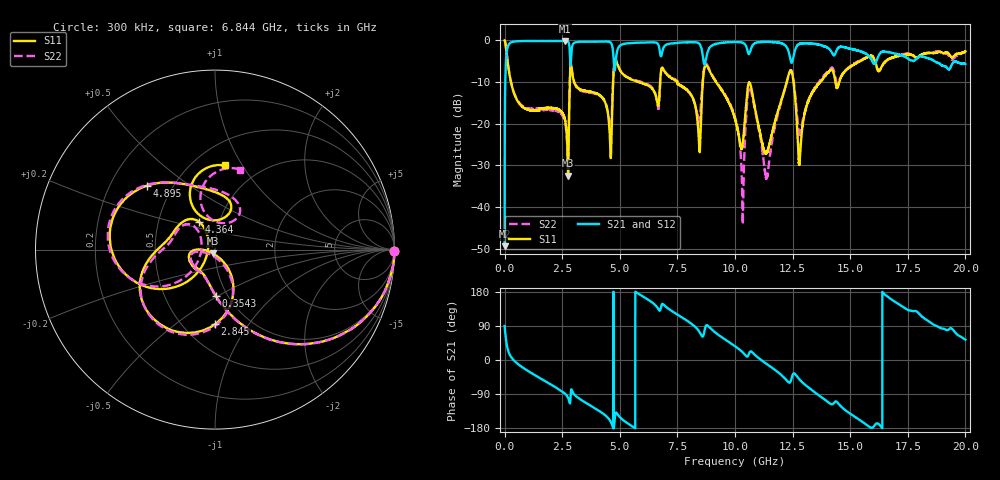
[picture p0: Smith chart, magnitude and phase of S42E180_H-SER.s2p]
!{S42E180}
!Johanson Technology Inc.
!www.johansontechnology.com
!Test Board Conditions:
!Substrate Type  RO4350B
!Substrate Thickness  50 mil
!Substrate Dk  3.66
!TL Type: GCPW
!TL Trace Width  60 mil
!TL Gap  10 mil
!Electrode orientation  Horizontal
!DUT TOPOLOGY	SERIES
!Mounting Pad LxW  14x55 mil
! Created Wed Nov 25 22:02:25 2020
# khz S ma R 50
! 2 Port Network Data from SP1.SP block
! freq  magS11  angS11  magS21  angS21  magS12  angS12  magS22  angS22
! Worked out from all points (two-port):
!   20001 points, 300 kHz to 20 GHz, reference 50 ohm
!   highest |S21| = -0.10 dB at 2.609 GHz (marker M1); lowest = -49.4 dB at 300 kHz (marker M2)
!   |S21| within 3 dB of the highest: 86.64 MHz to 2.834 GHz (2.747 GHz wide, 188 % of centre); 4.862 GHz to 6.751 GHz (1.889 GHz wide, 32.5 % of centre)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
!   lowest |S11| = -32.5 dB at 2.757 GHz (marker M3), VSWR 1.05, Z = 48.9 - j2.08 ohm
!   |S11| at or under -10 dB: 276.1 MHz to 2.831 GHz (2.555 GHz wide, 164 % of centre); 3.024 GHz to 4.71 GHz (1.687 GHz wide, 43.6 % of centre); 9.179 GHz to 12.25 GHz (3.066 GHz wide, 28.6 % of centre)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
!   |S22| runs from -44.2 to 0.0 dB; largest |S21 - S12| = 0.02
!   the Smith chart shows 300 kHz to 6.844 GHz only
!   S11 on the Smith chart (normalised r, x): 300 kHz: open; 354.3 MHz: 0.88, -0.49; 2.845 GHz: 0.71, -0.71; 4.364 GHz: 0.80, +0.26; 4.895 GHz: 0.36, +0.35; 6.844 GHz: 0.70, +0.84
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300  0.9996 -0.4  0.003383 89.9  0.003412 89.3  0.9975 -0.5
113300  0.6142 -56.2  0.7873 33.8  0.788 33.7  0.6156 -56.2
354300  0.259 -88.9  0.9609 2.1  0.9615 2.0  0.2611 -88.9
2609300  0.1153 -178.8  0.9885 -88.3  0.9878 -88.3  0.1073 -173.8
2757300  0.02377 -116.5  0.9662 -99.8  0.9667 -99.8  0.03878 -99.1
2845300  0.4162 -89.9  0.5899 -112.1  0.5907 -112.1  0.4301 -90.8
3334300  0.255 160.6  0.9651 -105.7  0.9635 -105.8  0.2484 167.8
4364300  0.1807 120.2  0.9714 -145.6  0.9716 -145.6  0.1813 132.5
4583300  0.05573 131.9  0.9531 -160.4  0.9513 -160.4  0.08027 158.3
4895300  0.5197 136.7  0.7677 -142.4  0.7674 -142.6  0.5252 136.9
6667300  0.1629 89.5  0.8979 135.1  0.8966 135.0  0.154 73.1
6844300  0.4716 83.5  0.7372 148.2  0.7367 148.1  0.4679 72.4
8159300  0.2065 2.3  0.9534 93.3  0.9502 93.5  0.2043 8.7
1.00003e7  0.1147 -44.8  0.9588 36.3  0.9591 36.3  0.1194 -57.7
1.03273e7  0.05533 21.3  0.9402 20.7  0.9398 20.7  0.009013 -43.0
1.06753e7  0.2926 -19.3  0.7637 22.5  0.7653 22.7  0.2583 -31.5
1.13693e7  0.04481 6.4  0.9609 -10.2  0.9612 -10.2  0.02219 158.8
1.23713e7  0.4192 1.4  0.6586 -59.9  0.6617 -59.8  0.4204 -8.5
1.27993e7  0.03255 -8.1  0.9086 -51.3  0.9077 -51.5  0.07403 -41.9
1.33343e7  0.2296 22.2  0.9138 -79.3  0.916 -79.1  0.2355 -5.8
1.66673e7  0.5952 -99.9  0.7258 165.4  0.7089 165.3  0.5931 -113.9
2e7  0.7376 155.2  0.5216 53.6  0.5242 54.6  0.7215 136.2
